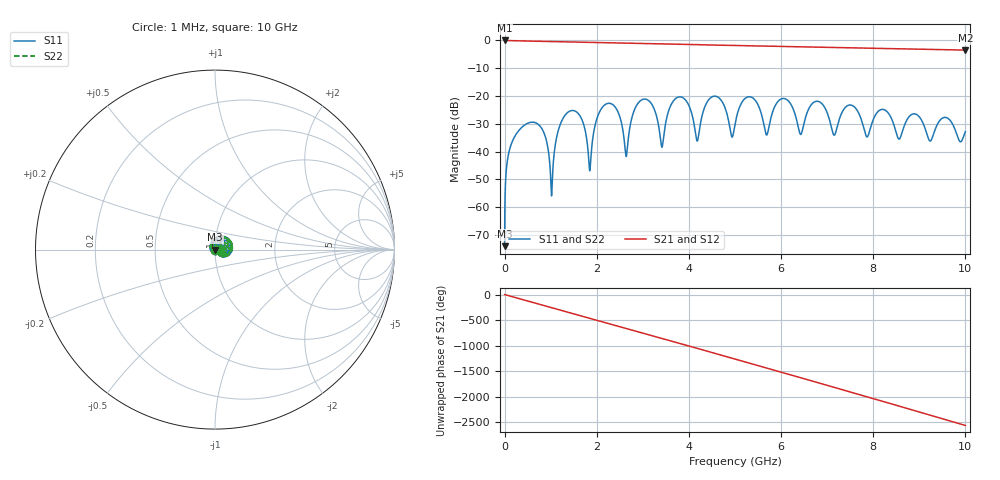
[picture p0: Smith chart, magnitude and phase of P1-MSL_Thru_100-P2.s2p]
!Created with skrf (http://scikit-rf.org).
# GHz S RI R 50.0
!freq ReS11 ImS11 ReS21 ImS21 ReS12 ImS12 ReS22 ImS22
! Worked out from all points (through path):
!   10000 points, 1 MHz to 10 GHz, reference 50 ohm
!   highest |S21| = 0.00 dB at 1 MHz (marker M1); lowest = -3.5 dB at 10 GHz (marker M2)
!   group delay of S21, straight-line fit = 711 ps
!   lowest |S11| = -74.0 dB at 1 MHz (marker M3), VSWR 1.00, Z = 50 - j0.0199 ohm
!   |S11| at or under -10 dB: start of sweep to end of sweep
!   |S22| runs from -74.0 to -20.0 dB; largest |S21 - S12| = 6.1e-16
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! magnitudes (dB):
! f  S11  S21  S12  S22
! 1 MHz  -74.0  0.0  0.0  -74.0
! 82 MHz  -41.2  0.0  0.0  -41.2
! 305 MHz  -32.5  -0.1  -0.1  -32.5
! 780 MHz  -31.0  -0.3  -0.3  -31.0
! 1.019 GHz  -55.9  -0.4  -0.4  -55.9
! 1.265 GHz  -28.1  -0.5  -0.5  -28.1
! 1.668 GHz  -28.1  -0.6  -0.6  -28.1
! 1.848 GHz  -46.9  -0.7  -0.7  -46.9
! 2.207 GHz  -22.8  -0.8  -0.8  -22.8
! 2.636 GHz  -41.7  -1.0  -1.0  -41.7
! 2.957 GHz  -21.6  -1.1  -1.1  -21.6
! 3.334 GHz  -29.9  -1.2  -1.2  -29.9
! 3.837 GHz  -20.4  -1.4  -1.4  -20.4
! 4.184 GHz  -36.2  -1.5  -1.5  -36.2
! 4.561 GHz  -20.0  -1.7  -1.7  -20.0
! 5.001 GHz  -30.1  -1.8  -1.8  -30.1
! 6.062 GHz  -20.9  -2.2  -2.2  -20.9
! 6.429 GHz  -33.8  -2.3  -2.3  -33.8
! 6.667 GHz  -22.9  -2.4  -2.4  -22.9
! 7.152 GHz  -34.1  -2.5  -2.5  -34.1
! 8.334 GHz  -26.3  -2.9  -2.9  -26.3
! 10 GHz  -32.8  -3.5  -3.5  -32.8
